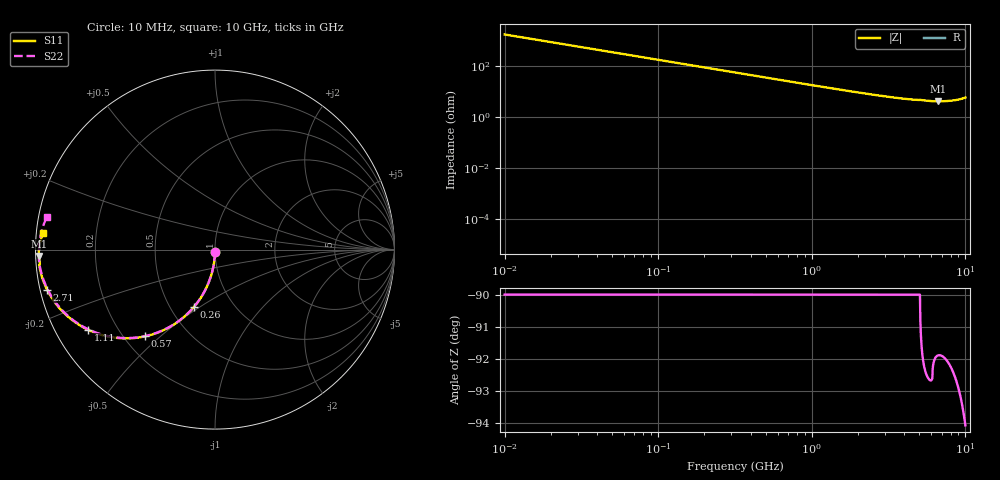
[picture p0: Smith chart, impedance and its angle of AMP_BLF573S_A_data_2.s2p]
! Created Mon Oct  5 10:26:43 2009
# ghz S ma R 50
! 2 Port Network Data from SP1.SP block
! freq  magS11  angS11  magS21  angS21  magS12  angS12  magS22  angS22
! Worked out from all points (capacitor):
!   1000 points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, 10 MHz to 10 GHz, reference 50 ohm
!   read as one part in shunt: C = 8.93 pF near 60 MHz
!   lowest |Z| = 4.16 ohm at 6.67 GHz (marker M1)
!   S11 on the Smith chart (normalised r, x): 10 MHz: 1.00, -0.03; 260 MHz: 0.65, -0.47; 570 MHz: 0.28, -0.45; 1.11 GHz: 0.10, -0.29; 2.71 GHz: 0.02, -0.12; 10 GHz: 0.02, +0.05
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0.01  0.01395 -90.8  0.9999 -0.8  0.9999 -0.8  0.01395 -90.8
0.04  0.05571 -93.2  0.9984 -3.2  0.9984 -3.2  0.05571 -93.2
0.07  0.09718 -95.6  0.9953 -5.6  0.9953 -5.6  0.09718 -95.7
0.09  0.1246 -97.2  0.9922 -7.2  0.9922 -7.2  0.1246 -97.3
0.11  0.1516 -98.8  0.9884 -8.8  0.9884 -8.8  0.1516 -98.8
0.17  0.2307 -103.5  0.973 -13.5  0.973 -13.5  0.2307 -103.5
0.26  0.3407 -110.1  0.9402 -20.2  0.9402 -20.2  0.3407 -110.2
0.39  0.4773 -118.8  0.8788 -28.9  0.8788 -28.9  0.4773 -119.0
0.57  0.621 -128.9  0.7838 -39.0  0.7838 -39.0  0.621 -129.0
0.83  0.7545 -139.7  0.6563 -49.8  0.6563 -49.8  0.7545 -139.9
1.11  0.8369 -147.8  0.5473 -57.9  0.5473 -57.9  0.8369 -148.1
1.37  0.8824 -153.1  0.4705 -63.3  0.4705 -63.3  0.8824 -153.5
1.68  0.9157 -157.8  0.4019 -68.0  0.4019 -68.0  0.9157 -158.3
2.13  0.9433 -162.5  0.332 -72.8  0.332 -72.8  0.9433 -163.2
2.71  0.9618 -166.6  0.2735 -77.0  0.2735 -77.0  0.9618 -167.5
3.34  0.9724 -169.6  0.2331 -80.2  0.2331 -80.2  0.9724 -170.8
4.24  0.98 -172.7  0.1989 -83.5  0.1989 -83.5  0.98 -174.2
5.01  0.9826 -174.9  0.1857 -85.9  0.1857 -85.9  0.9826 -176.9
6.09  0.9806 -176.8  0.1651 -90.5  0.1651 -90.5  0.976 -179.0
6.67  0.9823 -177.9  0.1641 -91.1  0.1641 -91.1  0.979 179.5
8.34  0.9786 178.9  0.1766 -95.5  0.1766 -95.5  0.9742 175.1
10  0.9619 174.6  0.2256 -102.4  0.2256 -102.4  0.9532 168.9
